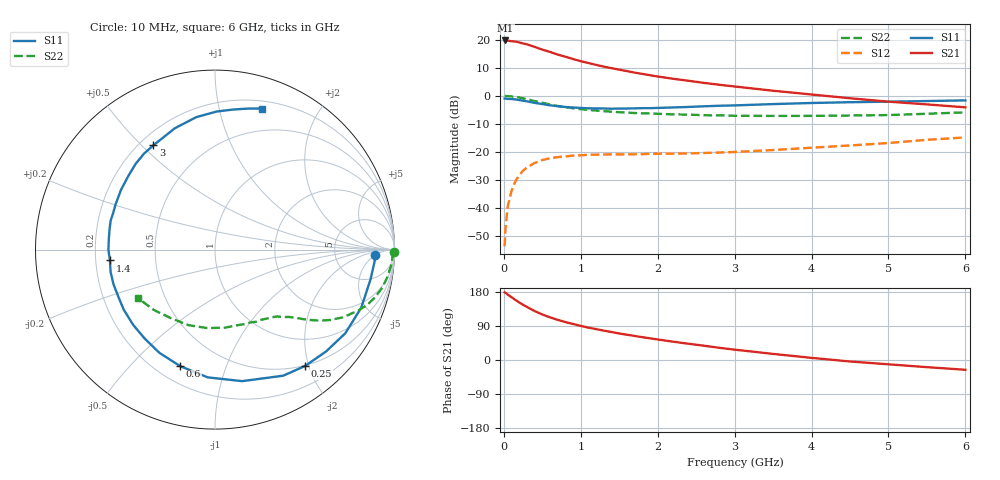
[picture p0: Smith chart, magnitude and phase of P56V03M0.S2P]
! SIEMENS Small Signal Semiconductors
! BFP183
! Si NPN RF Bipolar Junction Transistor in SOT143
! VCE = 6 V  IC = 3 mA
! Common Emitter S-Parameters:  March  1996
# GHz  S  MA  R  50
!  f  S11  S21  S12  S22
! GHz  MAG  ANG  MAG  ANG  MAG  ANG  MAG  ANG
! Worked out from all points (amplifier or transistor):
!   36 points, 10 MHz to 6 GHz, reference 50 ohm
!   highest |S21| = 19.7 dB at 20 MHz (marker M1)
!   |S21| within 3 dB of that: start of sweep to 472.4 MHz
!   unconditionally stable (mu >= 1): 1.921 GHz to 5.703 GHz
!   at 250 MHz: K = 0.15, MSG = 22.6 dB, |S12| = -26.7 dB
!   at 1.4 GHz: K = 0.77, MSG = 15.3 dB, |S12| = -20.9 dB
!   at 6 GHz: K = 0.94, MSG = 5.4 dB, |S12| = -14.8 dB
!   lowest NFmin = 1.10 dB at 450 MHz
!   S11 on the Smith chart (normalised r, x): 10 MHz: 16, -5; 250 MHz: 0.49, -1.94; 600 MHz: 0.29, -0.70; 1.4 GHz: 0.26, -0.05; 3 GHz: 0.25, +0.54; 6 GHz: 0.27, +1.36
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0.01  0.8942 -2.1  9.616 178.6  0.0021 83.3  0.9967 -0.9
0.02  0.8912 -4.5  9.682 177.6  0.0041 89.0  0.9899 -1.8
0.05  0.8821 -11.0  9.632 172.7  0.0106 86.9  0.988 -4.3
0.15  0.8628 -32.7  9.263 158.5  0.0299 71.8  0.9563 -12.8
0.2  0.8397 -42.5  8.935 151.9  0.0385 67.1  0.9312 -16.5
0.25  0.8198 -52.3  8.539 145.6  0.0465 62.1  0.9023 -20.0
0.3  0.7987 -61.6  8.261 140.1  0.053 57.6  0.8688 -22.9
0.4  0.7484 -78.3  7.438 129.1  0.0636 49.8  0.8068 -27.9
0.5  0.7131 -93.2  6.644 120.2  0.0718 43.3  0.751 -31.5
0.6  0.6777 -106.6  6.055 112.6  0.0775 38.2  0.7023 -34.3
0.7  0.6533 -118.3  5.425 106.0  0.0809 34.4  0.659 -36.5
0.8  0.6318 -128.3  4.972 100.0  0.0834 31.0  0.6268 -38.2
1  0.6088 -146.6  4.134 90.0  0.0872 26.0  0.5783 -40.9
1.1  0.5992 -154.1  3.838 85.3  0.0891 24.5  0.56 -42.1
1.4  0.5885 -174.1  3.105 73.8  0.0906 20.8  0.5222 -45.8
1.8  0.6034 164.5  2.456 60.2  0.0916 19.4  0.4879 -50.8
2.2  0.6205 147.5  2.013 48.3  0.0931 19.7  0.4672 -56.9
3  0.6749 120.6  1.466 27.3  0.1 22.8  0.441 -71.9
3.5  0.7123 108.3  1.232 16.1  0.1083 24.6  0.4382 -82.7
4.5  0.7693 89.3  0.905 -3.9  0.1305 25.2  0.4462 -109.4
5.5  0.8075 76.7  0.703 -18.9  0.1647 23.2  0.479 -135.5
6  0.8292 71.4  0.623 -25.8  0.1814 19.9  0.5078 -147.9
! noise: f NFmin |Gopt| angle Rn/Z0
0.45  1.1  0.37  35  0.3
0.9  1.15  0.34  85  0.23
1.8  1.9  0.35  160  0.13
